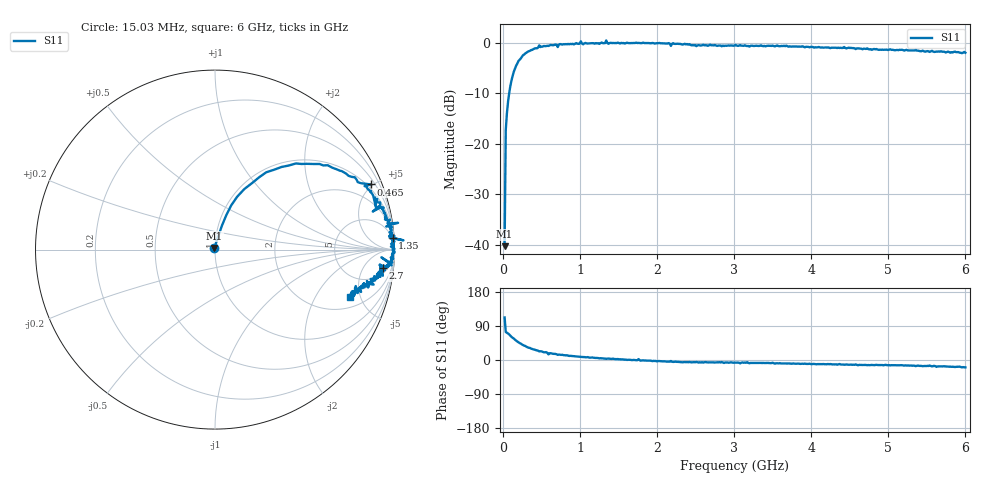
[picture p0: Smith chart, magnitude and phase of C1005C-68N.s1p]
!	Network	Analyzer	HP8753E.07.74:	Oct	30	2002	Serial	No.	JP38451487
!	Hewlett-Packard
!	28	Aug	2009	9:06:35
!	Frequency	S11
#	HZ	S	RI	R	50
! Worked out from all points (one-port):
!   400 points, 15.03 MHz to 6 GHz, reference 50 ohm
!   lowest |S11| = -40.2 dB at 15.03 MHz (marker M1), VSWR 1.02, Z = 49.6 + j0.894 ohm
!   |S11| at or under -10 dB: start of sweep to 74.44 MHz
!   S11 on the Smith chart (normalised r, x): 15.03 MHz: 0.99, +0.02; 465 MHz: 0.77, +4.87; 1.35 GHz: 4, +31; 2.7 GHz: 8, -14; 6 GHz: 2.78, -3.99
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1.502992e7  -0.0037 0.00901
3.002985e7  0.038 0.132
6.00297e7  0.0901 0.246
9.002955e7  0.163 0.337
1.95029e8  0.451 0.48
4.650277e8  0.868 0.363
5.550272e8  0.865 0.327
5.850271e8  0.897 0.236
6.150269e8  0.903 0.291
7.650262e8  0.929 0.229
9.750251e8  0.961 0.147
1.005025e9  1.02 0.149
1.035025e9  0.954 0.129
1.320023e9  0.988 0.0662
1.335023e9  1.05 0.0518
1.350023e9  0.99 0.0626
1.515022e9  0.981 0.0317
1.725021e9  1 -0.0101
1.755021e9  0.994 0.0426
1.785021e9  0.988 -0.03
2.175019e9  0.927 -0.0432
2.265019e9  0.972 -0.083
2.700016e9  0.935 -0.102
3.015015e9  0.943 -0.115
3.765011e9  0.904 -0.146
4.515007e9  0.869 -0.186
5.265004e9  0.811 -0.213
6e9  0.75 -0.264
